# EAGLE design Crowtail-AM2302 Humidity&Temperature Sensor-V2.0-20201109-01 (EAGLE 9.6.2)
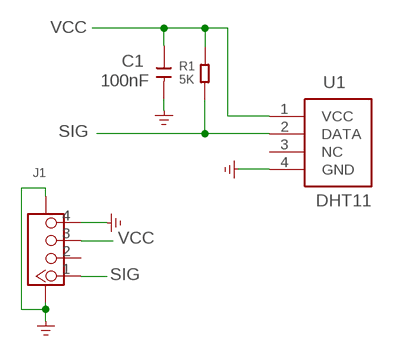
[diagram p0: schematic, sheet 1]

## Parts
C1  100nF  C0603  [0603]
J1  CONNECTOR_TWIG-4P-2.0-SMD-FEMALE-REINFORCE90D  [CONNECTOR_4P-SMD-2.0-90D]
R1  5K  R0603  [R0603]
U1  DHT11  [DHT11]

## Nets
GND: C1.2 J1.4 J1.SS1 J1.SS2 U1.4(GND)
SIG: J1.1 R1.1 U1.2(DATA)
VCC: C1.1 J1.3 R1.2 U1.1(VCC)
Unconnected: J1.2 U1.3(NC)

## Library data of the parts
C1 = A_xbj:C0603
J1 = A_xbj:CONNECTOR_TWIG-4P-2.0-SMD-FEMALE-REINFORCE
R1 = A_xbj:R0603
U1 = Sensors:DHT11

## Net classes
0 default: width 0.305 mm, drill 0.305 mm, clearance 0.305 mm

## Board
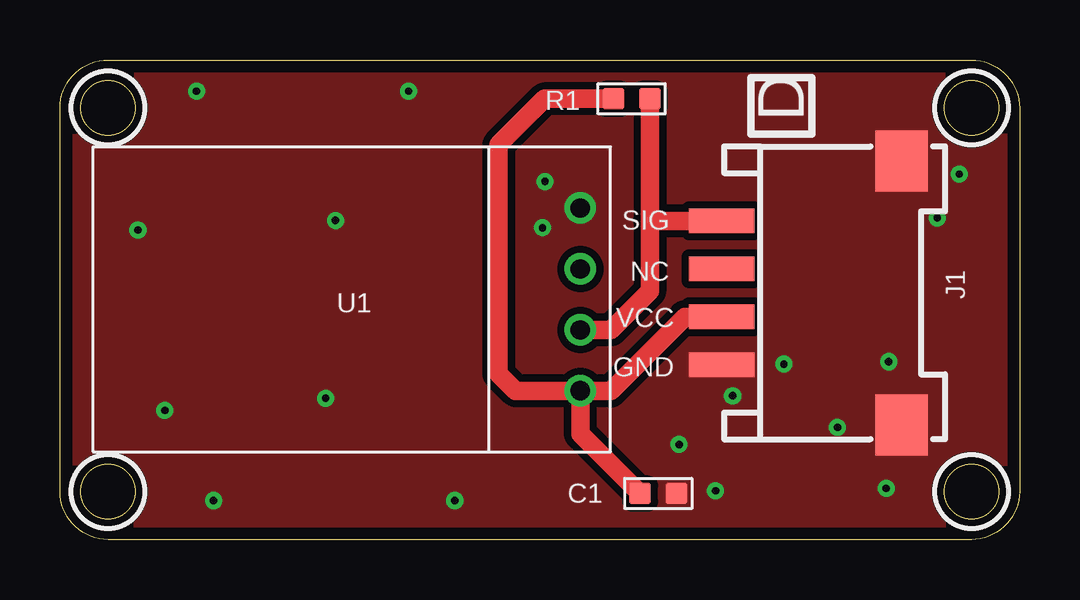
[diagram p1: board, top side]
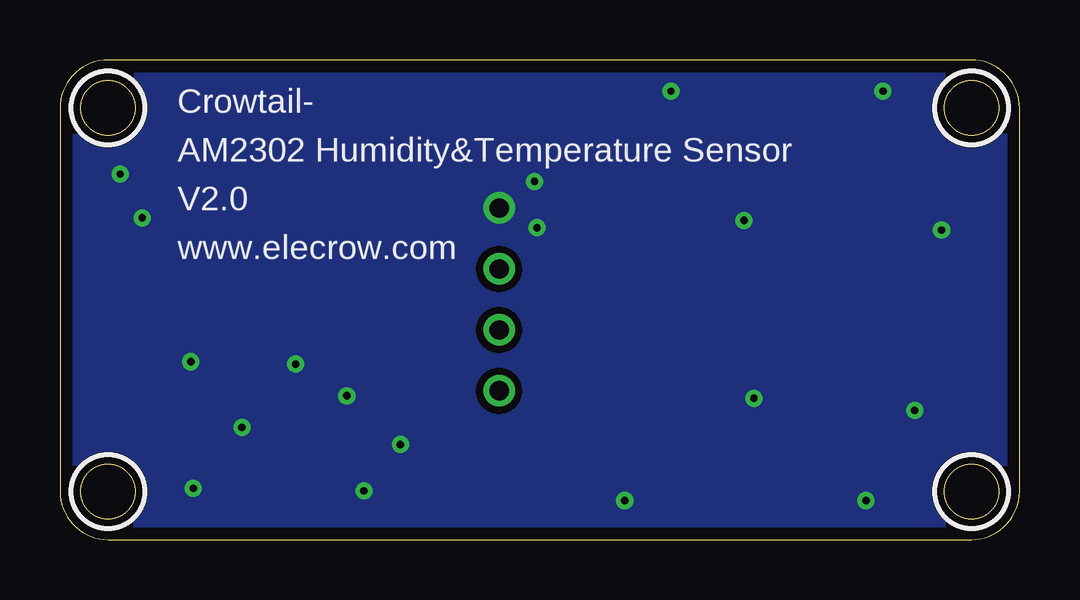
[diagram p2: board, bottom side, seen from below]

Size 40 x 20 mm. Coordinates in mm from the lower left corner, seen from the top.
Outline: 2,20 38,20 arc-90 40,18 40,2 arc-90 38,0 2,0 arc-90 0,2 0,18 arc-90 2,20
Outline: circle at 38,18 radius 1.14
Outline: circle at 38,2 radius 1.14
Outline: circle at 2,18 radius 1.14
Outline: circle at 2,2 radius 1.14
Copper layers (1*16): Top 0.035mm / dielectric 1.5mm / Bottom 0.035mm
Design rules "default *": minimum track width 10mil, minimum drill 10mil, track to track 8mil, track to pad 8mil, pad to pad 8mil, via to via 8mil, smd to smd 0mil, copper to edge 20mil, drill to drill 8mil, minimum pad ring 10mil, minimum via ring 8mil, stop-mask expansion 4mil, vias tented up to drill 100mil, thermal gap 10mil
tRestrict: area 36.5,16.5 to 39.5,19.5; area 36.5,0.5 to 39.5,3.5; area 0.5,16.5 to 3.5,19.5; area 0.5,0.5 to 3.5,3.5
bRestrict: area 36.5,16.5 to 39.5,19.5; area 36.5,0.5 to 39.5,3.5; area 0.5,16.5 to 3.5,19.5; area 0.5,0.5 to 3.5,3.5

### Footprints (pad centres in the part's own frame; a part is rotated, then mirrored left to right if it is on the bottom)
0603 = smd 0.889 x 0.889: 1 -0.762,0; 2 0.762,0
CONNECTOR_4P-SMD-2.0-90D = smd 1.01 x 2.74: 1 -3,-0.1; 2 -1,-0.1; 3 1,-0.1; 4 3,-0.1 | smd 2.54 x 2.184: SS1 -5.5,7.4; SS2 5.5,7.4
R0603 = smd 0.889 x 0.889: 1 -0.762,0; 2 0.762,0
DHT11 = drill 0.8: 1 -3.81,-3.81; 2 -1.27,-3.81; 3 1.27,-3.81; 4 3.81,-3.81

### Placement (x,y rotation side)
C1  24.94,1.92 0 top
J1  27.69,10.29 270 top
R1  23.83,18.38 180 top
U1  17.88,10.02 90 top

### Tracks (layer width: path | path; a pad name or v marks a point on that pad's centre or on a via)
GND  (via drill 0.3)
  other vias: 5.69,18.69 3.25,12.9 4.37,5.38 6.4,1.63 16.46,1.63 27.33,2.03 25.81,3.96 34.44,2.13 32.41,4.67 37.49,15.24 36.58,13.41 28.04,5.99 30.18,7.32 34.54,7.42 11.48,13.31 14.53,18.69 11.07,5.89 20.22,14.94 20.12,13
  pour Top (no thermals): 40.76,2.79 40.76,18.29 arc90 38.48,20.57 1.65,20.57 arc90 -0.64,18.29 -0.64,2.03 arc90 2.15,-0.76 37.21,-0.76 arc90
  pour Bottom (no thermals): 40.76,2.79 40.76,18.57 arc90 38.76,20.57 1.14,20.57 arc90 -0.64,18.8 -0.64,2.03 arc90 2.15,-0.76 37.21,-0.76 arc90
SIG
  Top 0.762: R1.1 24.59,13.31 | 24.59,13.31 24.59,10.36 22.97,8.74 U1.2 | J1.1 24.61,13.29 24.59,13.31
VCC
  Top 0.762: R1.2 20.2,18.38 18.29,16.46 18.29,6.91 18.99,6.21 U1.1 | J1.3 26.05,9.29 22.96,6.2 21.7,6.2 U1.1 | C1.1 21.69,4.41 U1.1

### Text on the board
tPlace: D | SIG | NC | VCC | GND
bPlace: Crowtail- | AM2302 Humidity&Temperature Sensor | V2.0 | www.elecrow.com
